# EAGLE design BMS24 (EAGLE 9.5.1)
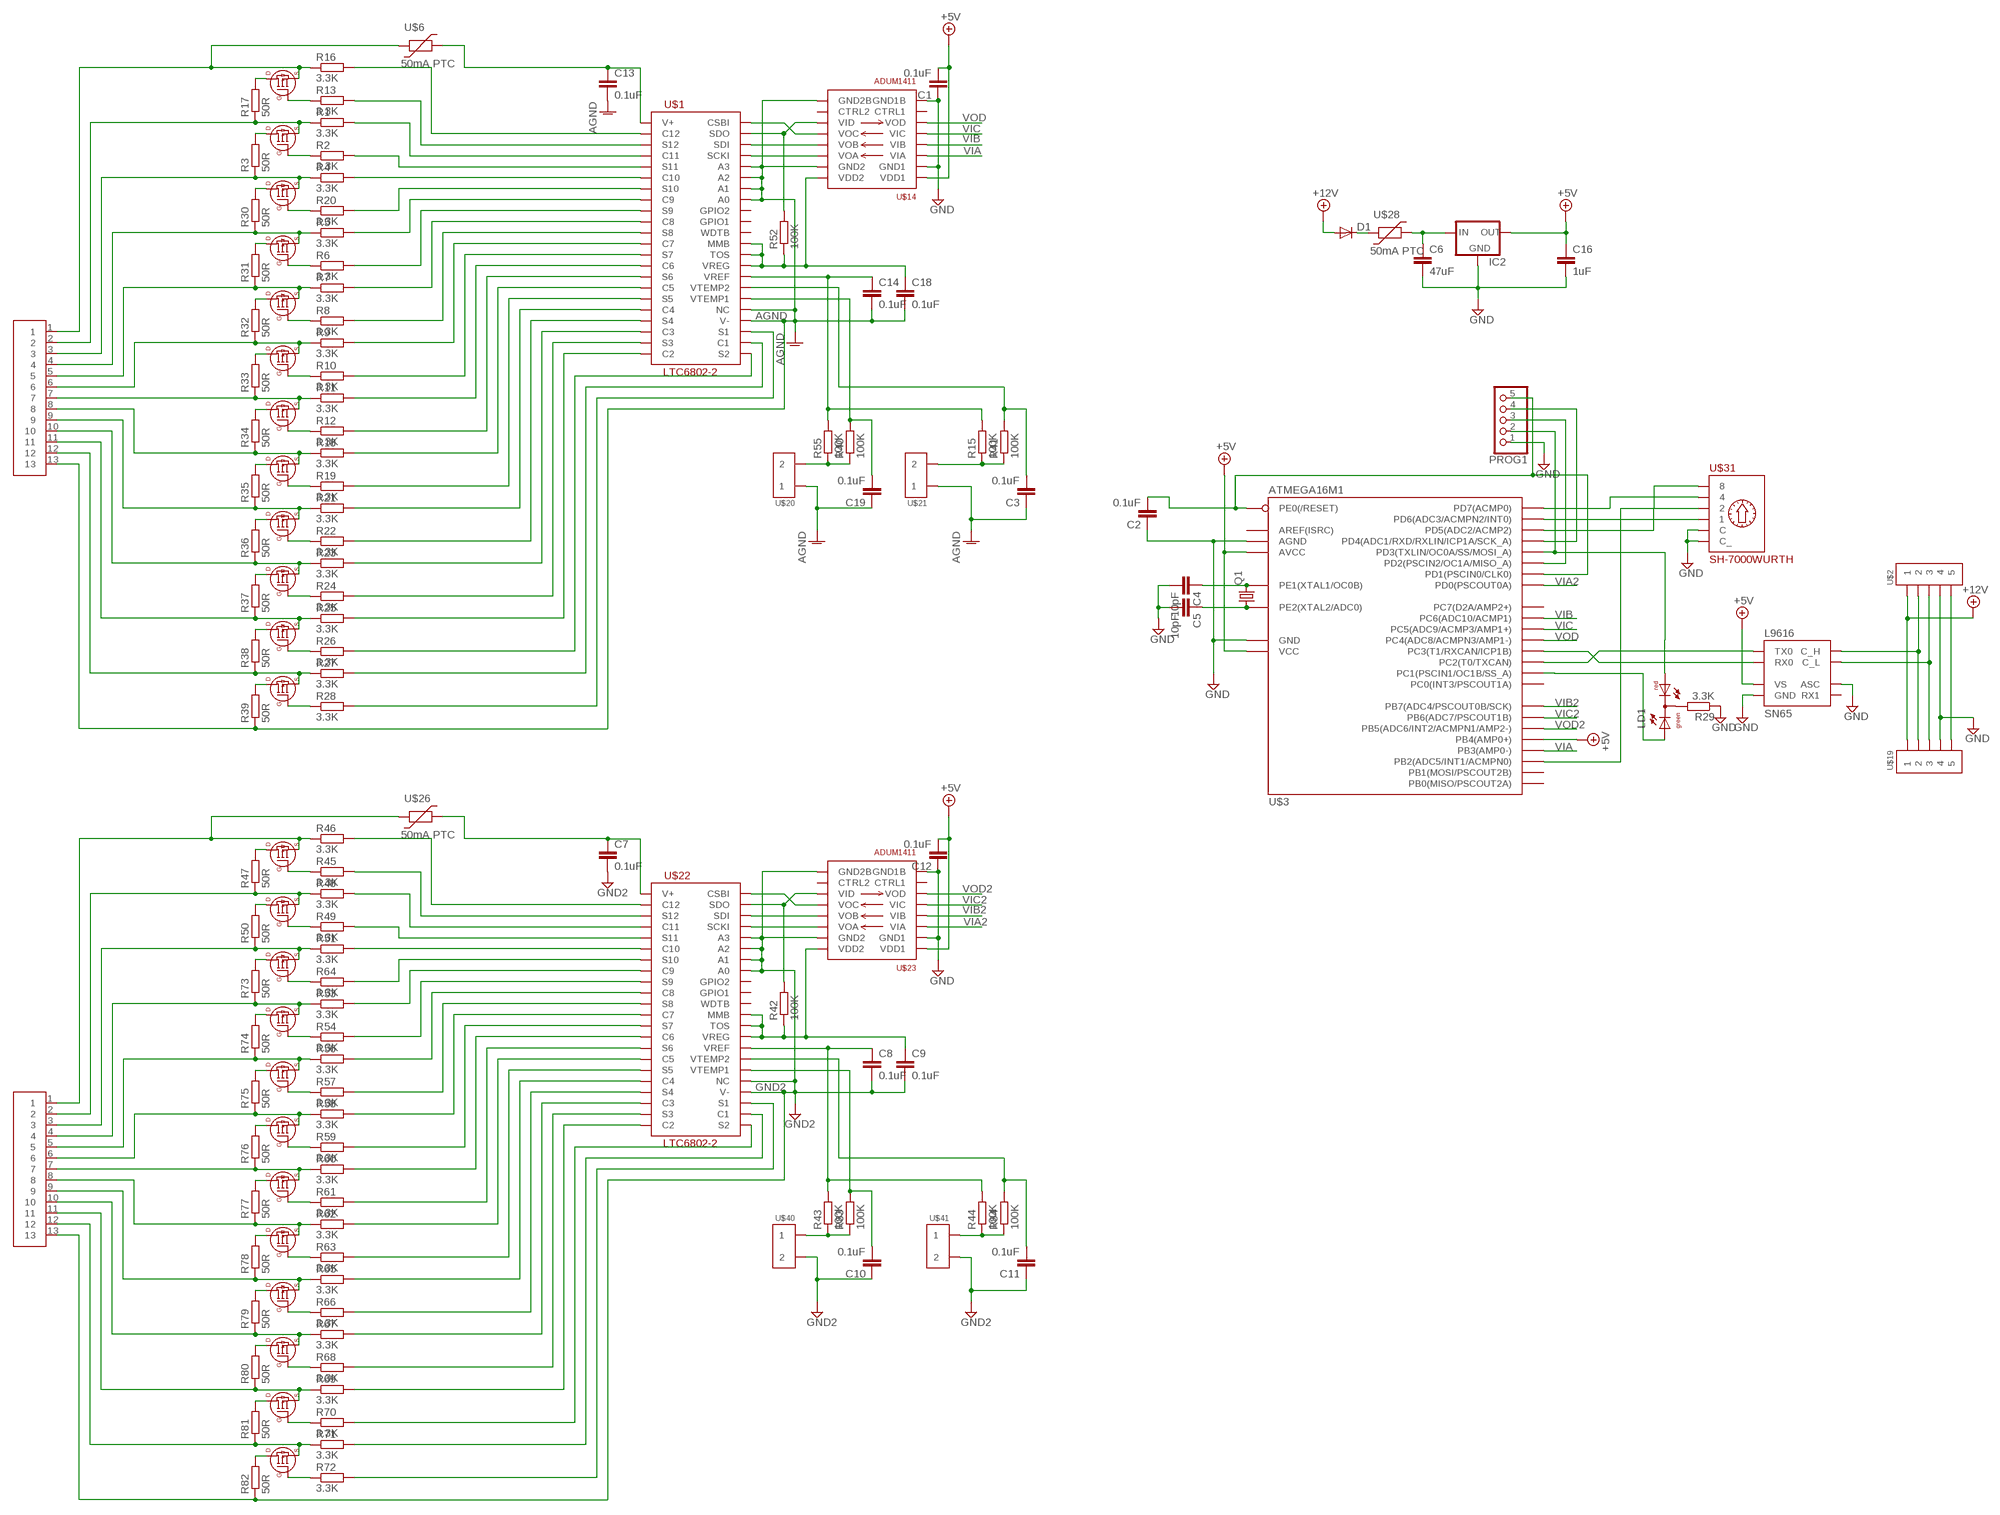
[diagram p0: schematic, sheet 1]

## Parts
C1  0.1uF  C-EUC0805  [C0805]
C2  0.1uF  C-EUC0805  [C0805]
C3  0.1uF  C-EUC0805  [C0805]
C4  10pF  C-EUC0805  [C0805]
C5  10pF  C-EUC0805  [C0805]
C6  47uF  C-EUC1206  [C1206]
C7  0.1uF  C-EUC0805  [C0805]
C8  0.1uF  C-EUC0805  [C0805]
C9  0.1uF  C-EUC0805  [C0805]
C10  0.1uF  C-EUC0805  [C0805]
C11  0.1uF  C-EUC0805  [C0805]
C12  0.1uF  C-EUC0805  [C0805]
C13  0.1uF  C-EUC0805  [C0805]
C14  0.1uF  C-EUC0805  [C0805]
C16  1uF  C-EUC0805  [C0805]
C18  0.1uF  C-EUC0805  [C0805]
C19  0.1uF  C-EUC0805  [C0805]
D1  DIODE-SOD123  [SOD123]
IC2  78LXXSOT89  [SOT89R]
LD1  DUOLED-RG-C  [DUOLED-C-5MM]
PROG1  PINHD-1X5  [1X05]
Q1  CRYSTALCTS406  [CTS406]
R1  3.3K  R-EU_R0805  [R0805]
R2  3.3K  R-EU_R0805  [R0805]
R3  50R  R-EU_R2512  [R2512]
R4  3.3K  R-EU_R0805  [R0805]
R5  3.3K  R-EU_R0805  [R0805]
R6  3.3K  R-EU_R0805  [R0805]
R7  3.3K  R-EU_R0805  [R0805]
R8  3.3K  R-EU_R0805  [R0805]
R9  3.3K  R-EU_R0805  [R0805]
R10  3.3K  R-EU_R0805  [R0805]
R11  3.3K  R-EU_R0805  [R0805]
R12  3.3K  R-EU_R0805  [R0805]
R13  3.3K  R-EU_R0805  [R0805]
R15  100K  R-EU_R0805  [R0805]
R16  3.3K  R-EU_R0805  [R0805]
R17  50R  R-EU_R2512  [R2512]
R18  3.3K  R-EU_R0805  [R0805]
R19  3.3K  R-EU_R0805  [R0805]
R20  3.3K  R-EU_R0805  [R0805]
R21  3.3K  R-EU_R0805  [R0805]
R22  3.3K  R-EU_R0805  [R0805]
R23  3.3K  R-EU_R0805  [R0805]
R24  3.3K  R-EU_R0805  [R0805]
R25  3.3K  R-EU_R0805  [R0805]
R26  3.3K  R-EU_R0805  [R0805]
R27  3.3K  R-EU_R0805  [R0805]
R28  3.3K  R-EU_R0805  [R0805]
R29  3.3K  R-EU_R0805  [R0805]
R30  50R  R-EU_R2512  [R2512]
R31  50R  R-EU_R2512  [R2512]
R32  50R  R-EU_R2512  [R2512]
R33  50R  R-EU_R2512  [R2512]
R34  50R  R-EU_R2512  [R2512]
R35  50R  R-EU_R2512  [R2512]
R36  50R  R-EU_R2512  [R2512]
R37  50R  R-EU_R2512  [R2512]
R38  50R  R-EU_R2512  [R2512]
R39  50R  R-EU_R2512  [R2512]
R40  100K  R-EU_R0805  [R0805]
R41  100K  R-EU_R0805  [R0805]
R42  100K  R-EU_R0805  [R0805]
R43  100K  R-EU_R0805  [R0805]
R44  100K  R-EU_R0805  [R0805]
R45  3.3K  R-EU_R0805  [R0805]
R46  3.3K  R-EU_R0805  [R0805]
R47  50R  R-EU_R2512  [R2512]
R48  3.3K  R-EU_R0805  [R0805]
R49  3.3K  R-EU_R0805  [R0805]
R50  50R  R-EU_R2512  [R2512]
R51  3.3K  R-EU_R0805  [R0805]
R52  100K  R-EU_R0805  [R0805]
R53  3.3K  R-EU_R0805  [R0805]
R54  3.3K  R-EU_R0805  [R0805]
R55  100K  R-EU_R0805  [R0805]
R56  3.3K  R-EU_R0805  [R0805]
R57  3.3K  R-EU_R0805  [R0805]
R58  3.3K  R-EU_R0805  [R0805]
R59  3.3K  R-EU_R0805  [R0805]
R60  3.3K  R-EU_R0805  [R0805]
R61  3.3K  R-EU_R0805  [R0805]
R62  3.3K  R-EU_R0805  [R0805]
R63  3.3K  R-EU_R0805  [R0805]
R64  3.3K  R-EU_R0805  [R0805]
R65  3.3K  R-EU_R0805  [R0805]
R66  3.3K  R-EU_R0805  [R0805]
R67  3.3K  R-EU_R0805  [R0805]
R68  3.3K  R-EU_R0805  [R0805]
R69  3.3K  R-EU_R0805  [R0805]
R70  3.3K  R-EU_R0805  [R0805]
R71  3.3K  R-EU_R0805  [R0805]
R72  3.3K  R-EU_R0805  [R0805]
R73  50R  R-EU_R2512  [R2512]
R74  50R  R-EU_R2512  [R2512]
R75  50R  R-EU_R2512  [R2512]
R76  50R  R-EU_R2512  [R2512]
R77  50R  R-EU_R2512  [R2512]
R78  50R  R-EU_R2512  [R2512]
R79  50R  R-EU_R2512  [R2512]
R80  50R  R-EU_R2512  [R2512]
R81  50R  R-EU_R2512  [R2512]
R82  50R  R-EU_R2512  [R2512]
R83  100K  R-EU_R0805  [R0805]
R84  100K  R-EU_R0805  [R0805]
SN65  L9616  [SOIC8]
U$1  LTC6802-2  [SSOP-44]
U$2  MOLEX-39502-1005  [MOLEX-39502-1005]
U$3  ATMEGA16M1  [TQFP32]
U$4  SI2351DS  [SOT23]
U$5  SI2351DS  [SOT23]
U$6  50mA PTC  1206_POLYSWITCH  [1206]
U$7  SI2351DS  [SOT23]
U$8  SI2351DS  [SOT23]
U$9  SI2351DS  [SOT23]
U$10  SI2351DS  [SOT23]
U$11  SI2351DS  [SOT23]
U$12  SI2351DS  [SOT23]
U$13  SI2351DS  [SOT23]
U$14  ADUM1411  [SOIC16W]
U$15  SI2351DS  [SOT23]
U$16  SI2351DS  [SOT23]
U$17  SI2351DS  [SOT23]
U$18  MOLEX_TERM_BLOCK_13  [MOLEX_TERM_BLOCK_13]
U$19  MOLEX-39502-1005  [MOLEX-39502-1005]
U$20  MOLEX-39502-1002  [MOLEX-39502-1002]
U$21  MOLEX-39502-1002  [MOLEX-39502-1002]
U$22  LTC6802-2  [SSOP-44]
U$23  ADUM1411  [SOIC16W]
U$24  SI2351DS  [SOT23]
U$25  SI2351DS  [SOT23]
U$26  50mA PTC  1206_POLYSWITCH  [1206]
U$27  SI2351DS  [SOT23]
U$28  50mA PTC  1206_POLYSWITCH  [1206]
U$29  SI2351DS  [SOT23]
U$30  SI2351DS  [SOT23]
U$31  SH-7000WURTH  [WS-ROTV]
U$32  SI2351DS  [SOT23]
U$33  SI2351DS  [SOT23]
U$34  SI2351DS  [SOT23]
U$35  SI2351DS  [SOT23]
U$36  SI2351DS  [SOT23]
U$37  SI2351DS  [SOT23]
U$38  SI2351DS  [SOT23]
U$39  MOLEX_TERM_BLOCK_13  [MOLEX_TERM_BLOCK_13]
U$40  MOLEX-39502-1002  [MOLEX-39502-1002]
U$41  MOLEX-39502-1002  [MOLEX-39502-1002]

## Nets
+5V: C1.2 C12.2 C16.1 IC2.2(OUT) SN65.P$3(VS) U$3.4(VCC) U$3.19(AVCC) U$3.24(PB4(AMP0+)) U$14.1(VDD1) U$23.1(VDD1)
+12V: D1.A U$2.1 U$19.1
AGND: C3.1 C13.2 C14.2 C18.2 C19.1 R39.1 U$1.26(V-) U$1.27(NC) U$1.37(A0) U$1.38(A1) U$1.39(A2) U$1.40(A3) U$14.9(GND2B) U$14.15(GND2) U$18.13 U$20.1 U$21.1
GND: C1.1 C2.1 C4.2 C5.2 C6.2 C12.1 C16.2 IC2.4(GND) PROG1.1 R29.1 SN65.P$2(GND) SN65.P$8(ASC) U$2.4 U$3.5(GND) U$3.20(AGND) U$14.2(GND1) U$14.8(GND1B) U$19.4 U$23.2(GND1) U$23.8(GND1B) U$31.C U$31.C2(C_)
GND2: C7.2 C8.2 C9.2 C10.1 C11.1 R82.1 U$22.26(V-) U$22.27(NC) U$22.37(A0) U$22.38(A1) U$22.39(A2) U$22.40(A3) U$23.9(GND2B) U$23.15(GND2) U$39.13 U$40.2 U$41.2
N$1: D1.C U$28.P$1
N$2: R16.2 U$1.2(C12)
N$3: R13.2 U$1.3(S12)
N$4: R3.2 U$5.P$3(D)
N$5: R1.2 U$1.4(C11)
N$6: R1.1 R17.1 U$5.P$2(S) U$18.2
N$7: U$1.42(SDI) U$14.13(VOB)
N$8: R3.1 R4.1 U$7.P$2(S) U$18.3
N$9: R4.2 U$1.6(C10)
N$10: R26.2 U$1.23(S2)
N$11: U$1.41(SCKI) U$14.14(VOA)
N$12: R27.2 U$1.24(C1)
N$13: R28.2 U$1.25(S1)
N$14: R2.2 U$1.5(S11)
N$15: R52.2 U$1.43(SDO) U$14.11(VID)
N$16: U$1.44(CSBI) U$14.12(VOC)
N$17: R2.1 U$5.P$1(G)
N$18: R30.2 U$7.P$3(D)
N$19: C2.2 PROG1.5 U$3.31(PE0(/RESET)) U$3.32(PD1(PSCIN0/CLK0))
N$20: C6.1 IC2.1(IN) U$28.P$2
N$21: R5.2 U$1.8(C9)
N$22: R7.2 U$1.10(C8)
N$23: R9.2 U$1.12(C7)
N$24: R11.2 U$1.14(C6)
N$25: C18.1 R52.1 U$1.31(VREG) U$1.32(TOS) U$1.33(MMB) U$14.16(VDD2)
N$26: R18.2 U$1.16(C5)
N$27: R21.2 U$1.18(C4)
N$28: R23.2 U$1.20(C3)
N$29: R25.2 U$1.22(C2)
N$30: U$3.16(PB2(ADC5/INT1/ACMPN0)) U$31.2
N$31: R5.1 R30.1 U$8.P$2(S) U$18.4
N$32: LD1.AR PROG1.2 U$3.2(PD3(TXLIN/OC0A/SS/MOSI_A))
N$33: PROG1.3 U$3.1(PD2(PSCIN2/OC1A/MISO_A))
N$34: PROG1.4 U$3.12(PD4(ADC1/RXD/RXLIN/ICP1A/SCK_A))
N$35: U$22.42(SDI) U$23.13(VOB)
N$36: SN65.P$4(RX0) U$3.7(PC3(T1/RXCAN/ICP1B))
N$37: SN65.P$1(TX0) U$3.6(PC2(T0/TXCAN))
N$38: SN65.P$7(C_H) U$2.2 U$19.2
N$39: SN65.P$6(C_L) U$2.3 U$19.3
N$40: LD1.C R29.2
N$41: LD1.AX(AG) U$3.3(PC1(PSCIN1/OC1B/SS_A))
N$42: U$3.15(PD7(ACMP0)) U$31.4
N$44: U$3.14(PD6(ADC3/ACMPN2/INT0)) U$31.1
N$45: U$3.13(PD5(ADC2/ACMP2)) U$31.8
N$46: C3.2 R41.2 U$1.29(VTEMP2)
N$47: U$2.5 U$19.5
N$48: C4.1 Q1.3 U$3.10(PE1(XTAL1/OC0B))
N$49: C5.1 Q1.1 U$3.11(PE2(XTAL2/ADC0))
N$50: R17.2 U$4.P$3(D)
N$51: R16.1 U$4.P$2(S) U$6.P$1 U$18.1
N$52: R13.1 U$4.P$1(G)
N$53: R7.1 R31.1 U$9.P$2(S) U$18.5
N$54: R31.2 U$8.P$3(D)
N$55: R6.1 U$8.P$1(G)
N$56: R20.1 U$7.P$1(G)
N$57: R8.1 U$9.P$1(G)
N$58: R10.1 U$10.P$1(G)
N$59: R12.1 U$11.P$1(G)
N$60: R28.1 U$17.P$1(G)
N$61: R19.1 U$12.P$1(G)
N$62: R22.1 U$13.P$1(G)
N$63: R24.1 U$15.P$1(G)
N$64: R26.1 U$16.P$1(G)
N$65: R27.1 R38.1 U$17.P$2(S) U$18.12
N$66: C14.1 R15.2 R55.2 U$1.30(VREF)
N$67: C19.2 R40.2 U$1.28(VTEMP1)
N$69: R25.1 R37.1 U$16.P$2(S) U$18.11
N$70: R23.1 R36.1 U$15.P$2(S) U$18.10
N$71: R38.2 U$16.P$3(D)
N$72: R39.2 U$17.P$3(D)
N$73: R37.2 U$15.P$3(D)
N$74: R21.1 R35.1 U$13.P$2(S) U$18.9
N$75: R36.2 U$13.P$3(D)
N$76: R18.1 R34.1 U$12.P$2(S) U$18.8
N$77: R35.2 U$12.P$3(D)
N$78: R11.1 R33.1 U$11.P$2(S) U$18.7
N$79: R9.1 R32.1 U$10.P$2(S) U$18.6
N$80: R33.2 U$10.P$3(D)
N$81: R34.2 U$11.P$3(D)
N$82: R32.2 U$9.P$3(D)
N$83: R24.2 U$1.21(S3)
N$84: R22.2 U$1.19(S4)
N$85: R40.1 R55.1 U$20.2
N$86: R15.1 R41.1 U$21.2
N$87: R20.2 U$1.7(S10)
N$88: R6.2 U$1.9(S9)
N$89: R8.2 U$1.11(S8)
N$90: R10.2 U$1.13(S7)
N$91: R12.2 U$1.15(S6)
N$92: U$22.41(SCKI) U$23.14(VOA)
N$93: R19.2 U$1.17(S5)
N$94: R42.2 U$22.43(SDO) U$23.11(VID)
N$95: U$22.44(CSBI) U$23.12(VOC)
N$96: C9.1 R42.1 U$22.31(VREG) U$22.32(TOS) U$22.33(MMB) U$23.16(VDD2)
N$97: C8.1 R43.2 R44.2 U$22.30(VREF)
N$98: C10.2 R83.2 U$22.28(VTEMP1)
N$99: R70.2 U$22.23(S2)
N$100: R71.2 U$22.24(C1)
N$101: R72.2 U$22.25(S1)
N$102: C11.2 R84.2 U$22.29(VTEMP2)
N$103: R47.2 U$24.P$3(D)
N$104: R45.1 U$24.P$1(G)
N$105: R46.1 U$24.P$2(S) U$26.P$1 U$39.1
N$106: R46.2 U$22.2(C12)
N$107: R45.2 U$22.3(S12)
N$108: R48.2 U$22.4(C11)
N$109: R47.1 R48.1 U$25.P$2(S) U$39.2
N$110: R50.2 U$25.P$3(D)
N$111: R50.1 R51.1 U$27.P$2(S) U$39.3
N$112: R51.2 U$22.6(C10)
N$113: R49.2 U$22.5(S11)
N$114: R49.1 U$25.P$1(G)
N$115: R73.2 U$27.P$3(D)
N$116: R53.2 U$22.8(C9)
N$117: R56.2 U$22.10(C8)
N$118: R58.2 U$22.12(C7)
N$119: R60.2 U$22.14(C6)
N$120: R62.2 U$22.16(C5)
N$121: R65.2 U$22.18(C4)
N$122: R67.2 U$22.20(C3)
N$123: R69.2 U$22.22(C2)
N$124: R53.1 R73.1 U$29.P$2(S) U$39.4
N$125: R56.1 R74.1 U$30.P$2(S) U$39.5
N$126: R74.2 U$29.P$3(D)
N$127: R54.1 U$29.P$1(G)
N$128: R64.1 U$27.P$1(G)
N$129: R57.1 U$30.P$1(G)
N$130: R59.1 U$32.P$1(G)
N$131: R61.1 U$33.P$1(G)
N$132: R72.1 U$38.P$1(G)
N$133: R63.1 U$34.P$1(G)
N$134: R66.1 U$35.P$1(G)
N$135: R68.1 U$36.P$1(G)
N$136: R70.1 U$37.P$1(G)
N$137: R71.1 R81.1 U$38.P$2(S) U$39.12
N$138: R69.1 R80.1 U$37.P$2(S) U$39.11
N$139: R67.1 R79.1 U$36.P$2(S) U$39.10
N$140: R81.2 U$37.P$3(D)
N$141: R82.2 U$38.P$3(D)
N$142: R80.2 U$36.P$3(D)
N$143: R65.1 R78.1 U$35.P$2(S) U$39.9
N$144: R79.2 U$35.P$3(D)
N$145: R62.1 R77.1 U$34.P$2(S) U$39.8
N$146: R78.2 U$34.P$3(D)
N$147: R60.1 R76.1 U$33.P$2(S) U$39.7
N$148: R58.1 R75.1 U$32.P$2(S) U$39.6
N$149: R76.2 U$32.P$3(D)
N$150: R77.2 U$33.P$3(D)
N$151: R75.2 U$30.P$3(D)
N$152: R64.2 U$22.7(S10)
N$153: R54.2 U$22.9(S9)
N$154: R57.2 U$22.11(S8)
N$155: R59.2 U$22.13(S7)
N$156: R61.2 U$22.15(S6)
N$157: R63.2 U$22.17(S5)
N$158: R66.2 U$22.19(S4)
N$159: R68.2 U$22.21(S3)
N$160: R43.1 R83.1 U$40.1
N$161: R44.1 R84.1 U$41.1
V+: C13.1 U$1.1(V+) U$6.P$2
V+1: C7.1 U$22.1(V+) U$26.P$2
VIA: U$3.23(PB3(AMP0-)) U$14.3(VIA)
VIA2: U$3.29(PD0(PSCOUT0A)) U$23.3(VIA)
VIB: U$3.22(PC6(ADC10/ACMP1)) U$14.4(VIB)
VIB2: U$3.28(PB7(ADC4/PSCOUT0B/SCK)) U$23.4(VIB)
VIC: U$3.18(PC5(ADC9/ACMP3/AMP1+)) U$14.5(VIC)
VIC2: U$3.27(PB6(ADC7/PSCOUT1B)) U$23.5(VIC)
VOD: U$3.17(PC4(ADC8/ACMPN3/AMP1-)) U$14.6(VOD)
VOD2: U$3.26(PB5(ADC6/INT2/ACMPN1/AMP2-)) U$23.6(VOD)
Unconnected: SN65.P$5(RX1) U$1.34(WDTB) U$1.35(GPIO1) U$1.36(GPIO2) U$3.8(PB0(MISO/PSCOUT2A)) U$3.9(PB1(MOSI/PSCOUT2B)) U$3.21(AREF(ISRC)) U$3.25(PC7(D2A/AMP2+)) U$3.30(PC0(INT3/PSCOUT1A)) U$14.7(CTRL1) U$14.10(CTRL2) U$22.34(WDTB) U$22.35(GPIO1) U$22.36(GPIO2) U$23.7(CTRL1) U$23.10(CTRL2)

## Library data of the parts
C1-C14 C16 C18 C19 = resistor:C-EU: CAPACITOR, European symbol
D1 = diode:DIODE-: DIODE
IC2 = v-reg:78LXX: VOLTAGE REGULATOR
LD1 = led:DUOLED-RG-C: DUO LED 2 colors (red/green), 5 mm, round, common Cathode www.ligitek.com or other producers.
PROG1 = pinhead:PINHD-1X5: PIN HEADER
Q1 = crystal:CRYSTAL: CRYSTAL
R1-R13 R15-R84 = resistor:R-EU_: RESISTOR, European symbol
SN65 = Ians parts:L9616
U$1 U$22 = Ians parts:LTC6802-2
U$2 U$19 = Ians parts:MOLEX-39502-1005
U$3 = Ians parts:ATMEGA16M1
U$4 U$5 U$7-U$13 U$15-U$17 U$24 U$25 U$27 U$29 U$30 U$32-U$38 = Ians parts:SI2351DS
U$6 U$26 U$28 = Ians parts:1206_POLYSWITCH
U$14 U$23 = Ians parts:ADUM1411
U$18 U$39 = Ians parts:MOLEX_TERM_BLOCK_13
U$20 U$21 U$40 U$41 = Ians parts:MOLEX-39502-1002
U$31 = Ians parts:SH-7000

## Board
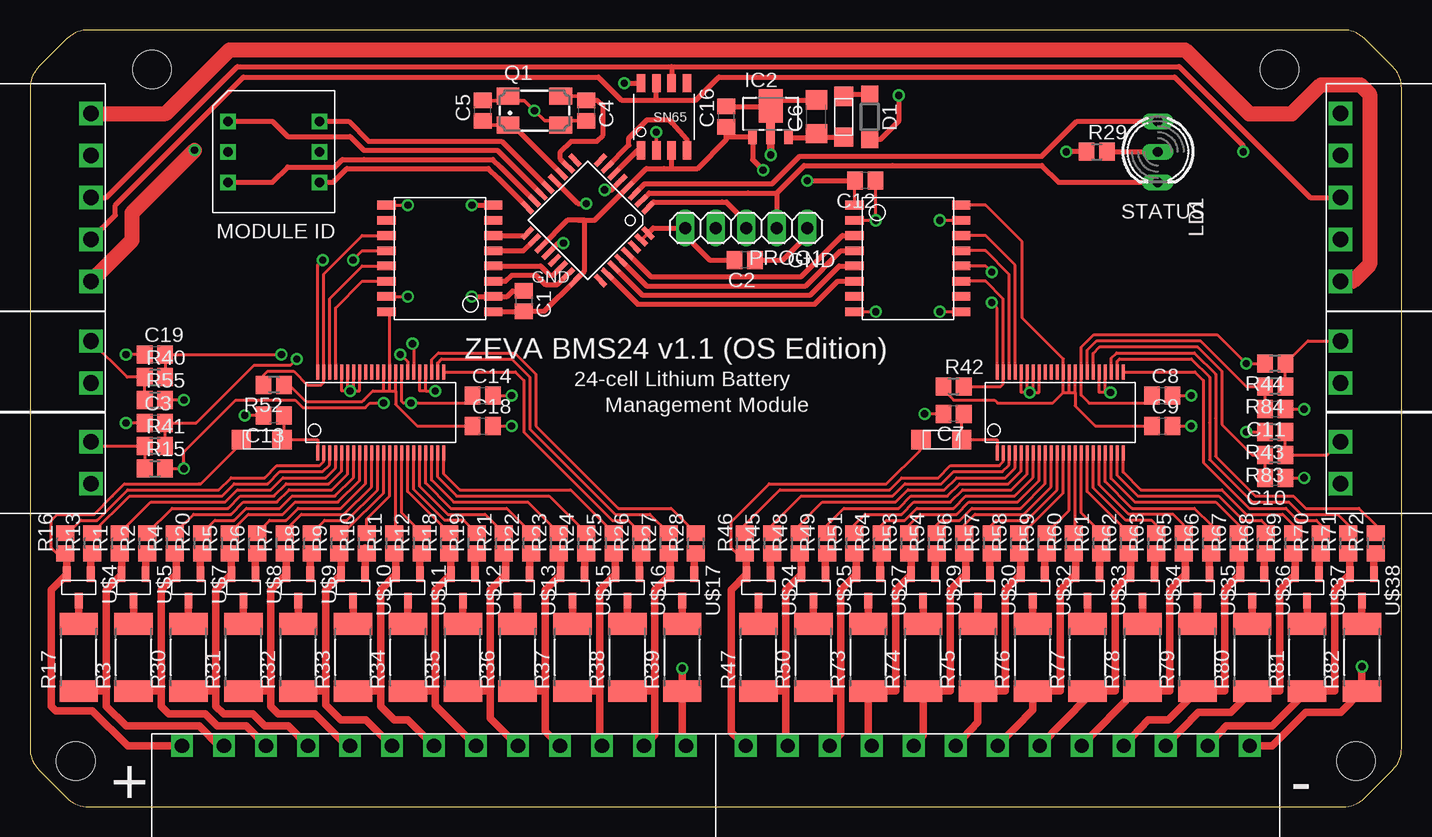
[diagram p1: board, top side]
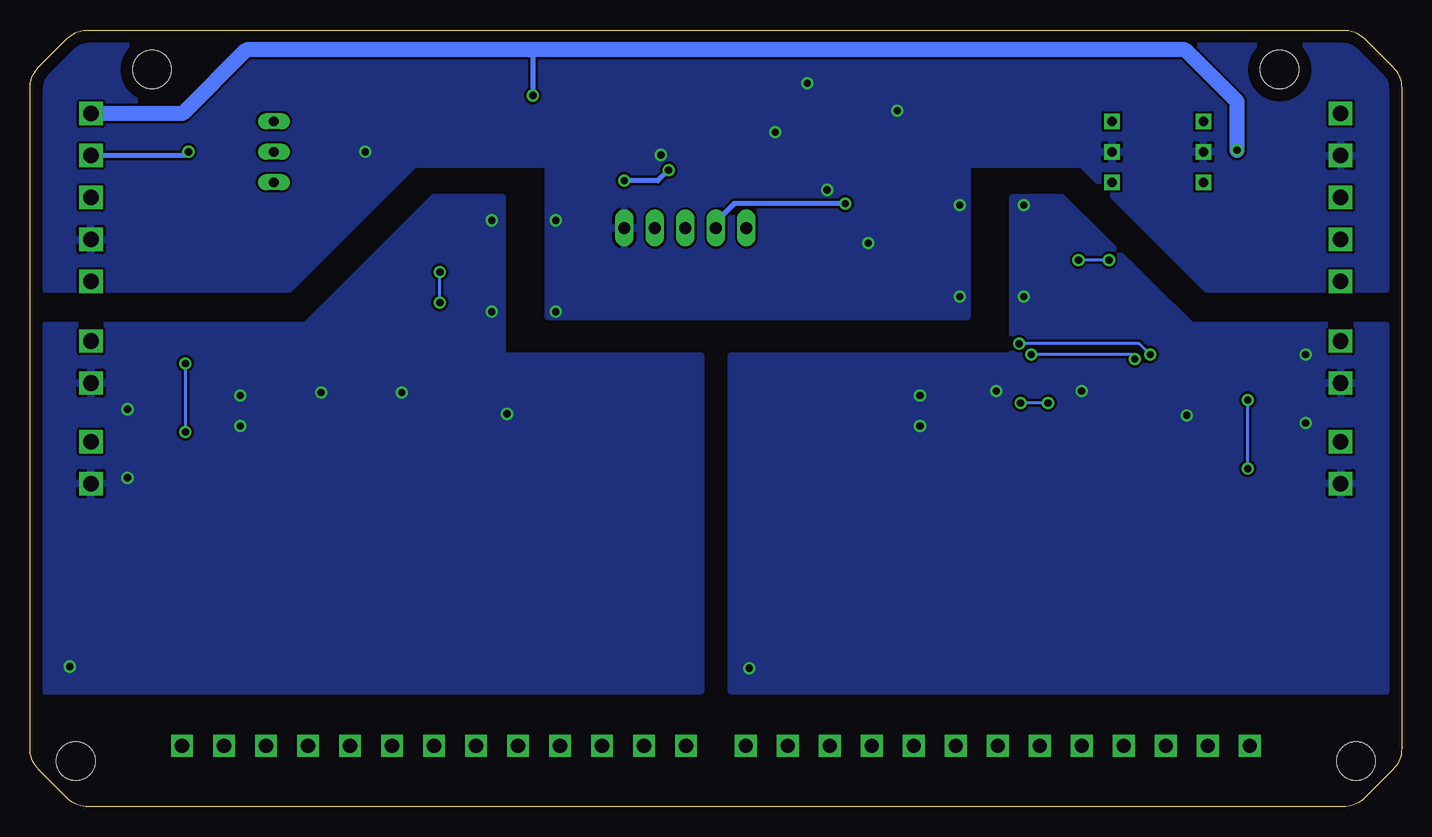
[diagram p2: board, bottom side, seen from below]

Size 114.3 x 64.77 mm. Coordinates in mm from the lower left corner, seen from the top.
Outline: 4.86,64.77 arc45 3.07,64.03 0.74,61.7 arc45 0,59.91 0,4.86 arc45 0.74,3.07 3.07,0.74 arc45 4.86,0 109.44,0 arc45 111.23,0.74 113.56,3.07 arc45 114.3,4.86 114.3,59.91 arc45 113.56,61.7 111.23,64.03 arc45 109.44,64.77 4.86,64.77
Copper layers (1*16): Top 0.035mm / dielectric 1.5mm / Bottom 0.035mm
Design rules "default *": minimum track width 10mil, minimum drill 10mil, track to track 8mil, track to pad 8mil, pad to pad 8mil, via to via 8mil, smd to smd 8mil, copper to edge 40mil, drill to drill 8mil, minimum pad ring 10mil, minimum via ring 8mil, stop-mask expansion 4mil, vias tented up to drill 0mil, thermal gap 10mil
Holes 3.2 mm at 3.81,3.81 110.49,3.81 10.16,61.47 104.14,61.47

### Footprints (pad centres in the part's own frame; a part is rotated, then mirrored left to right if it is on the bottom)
C0805 = smd 1.3 x 1.5: 1 -0.85,0; 2 0.85,0
C1206 = smd 1.6 x 1.8: 1 -1.4,0; 2 1.4,0
SOD123 = smd 1.4 x 1.4: A 1.9,0; C -1.9,0
SOT89R = smd 0.7 x 1.1: 1 1.5,-1.75; 2 -1.5,-1.75 | smd 0.7 x 1.8: 3 0,-1.4 | smd 2 x 2.8: 4 0,0.9
DUOLED-C-5MM = drill 0.813 long: AR 2.54,0; AX -2.54,0; C 0,0
1X05 = drill 1.016 long: 1 -5.08,0; 2 -2.54,0; 3 0,0; 4 2.54,0; 5 5.08,0
CTS406 = smd 1.9 x 1.4: 1 -2.2,-1.2; 2 2.2,-1.2; 3 2.2,1.2; 4 -2.2,1.2
R0805 = smd 1.3 x 1.5: 1 -0.85,0; 2 0.85,0
R2512 = smd 1.8 x 3.2: 1 -2.8,0; 2 2.8,0
SOIC8 = smd 1.524 x 0.711: P$1 -2.794,1.905; P$2 -2.794,0.635; P$3 -2.794,-0.635; P$4 -2.794,-1.905; P$5 2.794,-1.905; P$6 2.794,-0.635; P$7 2.794,0.635; P$8 2.794,1.905
SSOP-44 = smd 1.25 x 0.25: 1 -3.375,5.25; 2 -3.375,4.75; 3 -3.375,4.25; 4 -3.375,3.75; 5 -3.375,3.25; 6 -3.375,2.75; 7 -3.375,2.25; 8 -3.375,1.75; 9 -3.375,1.25; 10 -3.375,0.75; 11 -3.375,0.25; 12 -3.375,-0.25; 13 -3.375,-0.75; 14 -3.375,-1.25; 15 -3.375,-1.75; 16 -3.375,-2.25; 17 -3.375,-2.75; 18 -3.375,-3.25; 19 -3.375,-3.75; 20 -3.375,-4.25; 21 -3.375,-4.75; 22 -3.375,-5.25; 23 3.375,-5.25; 24 3.375,-4.75; 25 3.375,-4.25; 26 3.375,-3.75; 27 3.375,-3.25; 28 3.375,-2.75; 29 3.375,-2.25; 30 3.375,-1.75; 31 3.375,-1.25; 32 3.375,-0.75; 33 3.375,-0.25; 34 3.375,0.25; 35 3.375,0.75; 36 3.375,1.25; 37 3.375,1.75; 38 3.375,2.25; 39 3.375,2.75; 40 3.375,3.25; 41 3.375,3.75; 42 3.375,4.25; 43 3.375,4.75; 44 3.375,5.25
MOLEX-39502-1005 = drill 1.3 square: 1 -7,0; 2 -3.5,0; 3 0,0; 4 3.5,0; 5 7,0
TQFP32 = smd 1.2 x 0.4: 1 -4.3,2.8; 2 -4.3,2; 3 -4.3,1.2; 4 -4.3,0.4; 5 -4.3,-0.4; 6 -4.3,-1.2; 7 -4.3,-2; 8 -4.3,-2.8; 17 4.3,-2.8; 18 4.3,-2; 19 4.3,-1.2; 20 4.3,-0.4; 21 4.3,0.4; 22 4.3,1.2; 23 4.3,2; 24 4.3,2.8 | smd 0.4 x 1.2: 9 -2.8,-4.3; 10 -2,-4.3; 11 -1.2,-4.3; 12 -0.4,-4.3; 13 0.4,-4.3; 14 1.2,-4.3; 15 2,-4.3; 16 2.8,-4.3; 25 2.8,4.3; 26 2,4.3; 27 1.2,4.3; 28 0.4,4.3; 29 -0.4,4.3; 30 -1.2,4.3; 31 -2,4.3; 32 -2.8,4.3
SOT23 = smd 1.27 x 0.635: P$1 -1.1,1; P$2 -1.1,-1; P$3 1.1,0
1206 = smd 1.6 x 1.6: P$1 -1.7,0; P$2 1.7,0
SOIC16W = smd 1.524 x 0.711: 1 -4.445,4.445; 2 -4.445,3.175; 3 -4.445,1.905; 4 -4.445,0.635; 5 -4.445,-0.635; 6 -4.445,-1.905; 7 -4.445,-3.175; 8 -4.445,-4.445; 9 4.445,-4.445; 10 4.445,-3.175; 11 4.445,-1.905; 12 4.445,-0.635; 13 4.445,0.635; 14 4.445,1.905; 15 4.445,3.175; 16 4.445,4.445
MOLEX_TERM_BLOCK_13 = drill 1.2 square: 1 -21,0; 2 -17.5,0; 3 -14,0; 4 -10.5,0; 5 -7,0; 6 -3.5,0; 7 0,0; 8 3.5,0; 9 7,0; 10 10.5,0; 11 14,0; 12 17.5,0; 13 21,0
MOLEX-39502-1002 = drill 1.3 square: 1 -1.75,0; 2 1.75,0
WS-ROTV = drill 0.8 square: 1 -3.81,2.54; 2 3.81,-2.54; 4 -3.81,-2.54; 8 3.81,2.54; C -3.81,0; C2 3.81,0

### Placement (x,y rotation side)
C1  41.15,42.16 270 top
C2  59.56,45.59 180 top
C3  10.41,32 0 top
C4  46.35,58.04 270 top
C5  37.72,58.04 90 top
C6  65.53,57.53 90 top
C7  76.96,32.77 180 top
C8  94.36,34.29 0 top
C9  94.36,31.75 0 top
C10  103.76,27.43 180 top
C11  103.76,33.15 180 top
C12  69.6,52.2 180 top
C13  20.32,32.64 180 top
C14  37.72,34.29 0 top
C16  58.04,57.53 90 top
C18  37.72,31.75 0 top
C19  10.41,37.72 0 top
D1  69.98,57.53 270 top
IC2  61.72,57.53 0 top
LD1  93.98,54.61 270 top
PROG1  59.69,48.26 180 top
Q1  42.04,58.04 0 top
R1  7.49,21.97 90 top
R2  9.78,21.97 90 top
R3  8.64,12.45 90 top
R4  12.06,21.97 90 top
R5  16.64,21.97 90 top
R6  18.92,21.97 90 top
R7  21.21,21.97 90 top
R8  23.5,21.97 90 top
R9  25.78,21.97 90 top
R10  28.07,21.97 90 top
R11  30.35,21.97 90 top
R12  32.64,21.97 90 top
R13  5.21,21.97 90 top
R15  10.41,28.19 0 top
R16  2.92,21.97 90 top
R17  4.06,12.45 90 top
R18  34.92,21.97 90 top
R19  37.21,21.97 90 top
R20  14.35,21.97 90 top
R21  39.5,21.97 90 top
R22  41.78,21.97 90 top
R23  44.07,21.97 90 top
R24  46.35,21.97 90 top
R25  48.64,21.97 90 top
R26  50.93,21.97 90 top
R27  53.21,21.97 90 top
R28  55.5,21.97 90 top
R29  88.9,54.61 0 top
R30  13.21,12.45 90 top
R31  17.78,12.45 90 top
R32  22.35,12.45 90 top
R33  26.92,12.45 90 top
R34  31.5,12.45 90 top
R35  36.07,12.45 90 top
R36  40.64,12.45 90 top
R37  45.21,12.45 90 top
R38  49.78,12.45 90 top
R39  54.36,12.45 90 top
R40  10.41,35.81 0 top
R41  10.41,30.1 0 top
R42  76.96,35.05 0 top
R43  103.76,31.24 180 top
R44  103.76,36.96 180 top
R45  61.85,21.97 90 top
R46  59.56,21.97 90 top
R47  60.71,12.45 90 top
R48  64.14,21.97 90 top
R49  66.42,21.97 90 top
R50  65.28,12.45 90 top
R51  68.71,21.97 90 top
R52  20.32,35.18 180 top
R53  73.28,21.97 90 top
R54  75.56,21.97 90 top
R55  10.41,33.91 0 top
R56  77.85,21.97 90 top
R57  80.14,21.97 90 top
R58  82.42,21.97 90 top
R59  84.71,21.97 90 top
R60  87,21.97 90 top
R61  89.28,21.97 90 top
R62  91.57,21.97 90 top
R63  93.85,21.97 90 top
R64  70.99,21.97 90 top
R65  96.14,21.97 90 top
R66  98.42,21.97 90 top
R67  100.71,21.97 90 top
R68  103,21.97 90 top
R69  105.28,21.97 90 top
R70  107.57,21.97 90 top
R71  109.86,21.97 90 top
R72  112.14,21.97 90 top
R73  69.85,12.45 90 top
R74  74.42,12.45 90 top
R75  78.99,12.45 90 top
R76  83.57,12.45 90 top
R77  88.14,12.45 90 top
R78  92.71,12.45 90 top
R79  97.28,12.45 90 top
R80  101.85,12.45 90 top
R81  106.43,12.45 90 top
R82  111,12.45 90 top
R83  103.76,29.34 180 top
R84  103.76,35.05 180 top
SN65  52.83,57.53 90 top
U$1  29.21,32.89 90 top
U$2  5.08,50.8 90 top
U$3  46.48,48.9 225 top
U$4  4.06,18.29 270 top
U$5  8.64,18.29 270 top
U$6  19.3,30.61 0 top
U$7  13.21,18.29 270 top
U$8  17.78,18.29 270 top
U$9  22.35,18.29 270 top
U$10  26.92,18.29 270 top
U$11  31.5,18.29 270 top
U$12  36.07,18.29 270 top
U$13  40.64,18.29 270 top
U$14  34.16,45.72 180 top
U$15  45.21,18.29 270 top
U$16  49.78,18.29 270 top
U$17  54.36,18.29 270 top
U$18  33.66,5.08 0 top
U$19  109.22,50.8 270 top
U$20  5.08,37.08 90 top
U$21  5.08,28.7 90 top
U$22  85.85,32.89 90 top
U$23  73.15,45.72 0 top
U$24  60.71,18.29 270 top
U$25  65.28,18.29 270 top
U$26  75.95,30.61 0 top
U$27  69.85,18.29 270 top
U$28  67.82,57.53 270 top
U$29  74.42,18.29 270 top
U$30  78.99,18.29 270 top
U$31  20.32,54.61 0 top
U$32  83.57,18.29 270 top
U$33  88.14,18.29 270 top
U$34  92.71,18.29 270 top
U$35  97.28,18.29 270 top
U$36  101.85,18.29 270 top
U$37  106.43,18.29 270 top
U$38  111,18.29 270 top
U$39  80.64,5.08 0 top
U$40  109.22,28.7 270 top
U$41  109.22,37.08 270 top

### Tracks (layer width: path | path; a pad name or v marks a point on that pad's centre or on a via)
+5V  (via drill 0.6)
  Top 0.254: U$23.1 68.71,52.16 C12.2
  Top 0.406: U$14.1 41.11,41.27 C1.2 42.86,41.31 U$3.24 46.23,44.68 46.23,47.24 46.23,48.9 45.72,48.9 | U$3.19 44.78,48.9 45.72,48.9 | 45.72,48.9 45.85,48.9 47.05,48.9 U$3.4 51.37,53.21 52.83,53.21 | 52.83,53.21 55.63,53.21 58.04,55.63 58.04,55.88 | 58.04,55.88 C16.1 | SN65.P$3 53.47,53.21 52.83,53.21 | 58.04,55.88 60.22,55.88 IC2.2 60.22,53.95 v61.09,53.09 | v64.77,52.2 C12.2
  Bottom 0.406: v64.77,52.2 61.98,52.2 v61.09,53.09
+12V  (via drill 0.6)
  Top 0.406: D1.A 70.87,55.63 72.39,57.15 v72.39,59.31
  Top 1.27: U$2.1 8.51,47.23 8.51,49.53 v13.72,54.74
  Bottom 0.406: v72.39,59.31 72.39,63.12 72.64,63.12
  Bottom 1.27: U$19.1 101.58,57.8 96.27,63.12 72.64,63.12 18.03,63.12 13.72,58.8 v13.72,54.74
AGND  (via drill 0.6)
  Top 0.254: 32.96,34.67 U$1.26 | 32.96,34.67 v33.78,34.67 | U$1.27 32.46,34.67 32.96,34.67 | U$1.37 27.46,34.67 v26.67,34.67 | U$1.38 26.96,34.67 v26.67,34.67 | U$1.39 26.46,34.67 v26.67,34.67 | U$1.40 25.96,34.67 v26.67,34.67 | C14.2 v40.13,34.29 | C18.2 v40.13,31.75 | C3.1 v8,32 | C19.1 v8,37.72 | C13.2 v17.91,32.64 | U$14.15 v31.5,42.55 | U$14.9 v31.5,50.16
  Top 0.61: v54.36,11.56 R39.1 54.36,5.38 U$18.13
  pour Bottom: 1.27,9.65 55.88,9.65 55.88,37.59 32.38,37.59 32.38,50.8 28.32,50.8 17.53,40.13 1.27,40.13
GND  (via drill 0.6)
  Top 0.254: U$23.2 v70.48,48.9 70.48,52.16 C12.1 | U$23.8 v70.48,41.27
  Top 0.305: SN65.P$2 v52.2,56.26 | C5.2 41.19,58.89 v42.04,58.04 42.89,57.19 C4.2
  Top 0.406: C1.1 40.22,43.01 39.75,42.55 U$14.2 v36.83,42.55 | v36.83,50.16 U$14.8 | U$3.20 44.01,46.99 v44.45,46.99 | v47.88,51.44 48.46,51.44 U$3.5 | C2.1 62.74,45.59 64.77,47.62 PROG1.1 | v49.53,60.33 SN65.P$8 | C6.2 62.22,58.93 IC2.4 61.67,58.38 C16.2 | R29.1 v86.36,54.61
  Top 0.61: IC2.4 v61.72,54.36
  pour Bottom: 36.2,40.89 36.2,53.59 26.67,53.59 16.26,43.18 1.27,43.18 1.27,63.5 113.03,63.5 113.03,43.18 92.71,43.18 82.3,53.59 71.12,53.59 71.12,40.89
GND2  (via drill 0.6)
  Top 0.254: U$22.39 83.1,34.54 v83.31,34.54 | U$22.40 82.6,34.54 v83.31,34.54 | U$22.38 83.6,34.54 v83.31,34.54 | U$22.37 84.1,34.54 v83.31,34.54 | C8.2 v96.77,34.29 | C9.2 v96.77,31.75 | U$22.26 89.6,34.54 v90.04,34.54 89.1,34.54 U$22.27 | C10.1 v106.17,27.43 | C11.1 v106.17,33.15 | C7.2 v74.55,32.77 | v75.82,41.27 U$23.9 | v75.82,48.9 U$23.15
  Top 0.61: v111,11.68 R82.1 109.23,7.87 106.3,7.87 103.5,5.08 U$39.13
  pour Bottom: 58.42,9.65 113.03,9.65 113.03,40.13 91.31,40.13 80.64,50.8 74.93,50.8 74.93,37.59 58.42,37.59
N$1
  Top 0.406: D1.C 68.02,59.43 U$28.P$1
N$2
  Top 0.254: U$1.2 24.46,28.78 24.13,28.45 20.57,28.45 19.56,27.43 16.76,27.43 15.75,26.42 8.13,26.42 5.59,23.88 4.23,23.88 3.17,22.82 R16.2
N$3
  Top 0.254: U$1.3 24.96,28.52 24.38,27.94 20.83,27.94 19.81,26.92 17.02,26.92 16,25.91 8.29,25.91 R13.2
N$4
  Top 0.61: R3.2 U$5.P$3
N$5
  Top 0.254: U$1.4 25.46,28.25 24.64,27.43 21.08,27.43 20.07,26.42 17.27,26.42 16.26,25.4 10.07,25.4 R1.2
N$6
  Top 0.61: 6.35,9.65 6.35,18.1 U$5.P$2 7.64,20.98 R1.1 | R17.1 6.35,9.65 | 6.35,9.65 6.35,8.38 8,6.73 8.38,6.73 14.1,6.73 15.75,5.08 U$18.2
N$7
  Top 0.254: U$1.42 24.96,42.36 27.69,45.09 U$14.13
N$8
  Top 0.61: 10.92,9.65 10.92,18.1 U$7.P$2 12.21,20.98 R4.1 | R3.1 10.92,9.65 | U$18.3 18,6.73 15.62,6.73 14.61,7.75 11.56,7.75 10.92,8.38 10.92,9.65
N$9
  Top 0.254: U$1.6 26.46,27.73 25.15,26.42 21.59,26.42 20.57,25.4 17.78,25.4 16.76,24.38 13.63,24.38 R4.2
N$10
  Top 0.254: U$1.23 40.44,36.27 41.15,35.56 41.15,31.24 48.51,23.88 49.87,23.88 R26.2
N$11
  Top 0.254: U$1.41 25.46,41.59 27.69,43.81 U$14.14
N$12
  Top 0.254: U$1.24 33.96,37.01 34.29,37.34 40.13,37.34 41.66,35.81 41.66,31.5 48.77,24.38 51.65,24.38 R27.2
N$13
  Top 0.254: U$1.25 33.46,37.27 34.04,37.85 40.39,37.85 42.16,36.07 42.16,31.75 49.02,24.89 53.43,24.89 R28.2
N$14
  Top 0.254: U$1.5 25.96,27.99 24.89,26.92 21.34,26.92 20.32,25.91 17.53,25.91 16.51,24.89 11.85,24.89 R2.2
N$15
  Top 0.254: R52.2 19.47,35.98 19.81,36.32 21.97,36.32 23.11,35.18 24.26,35.18 24.46,35.38 U$1.43 24.46,44.4 27.69,47.62 U$14.11
N$16  (via drill 0.6)
  Top 0.254: U$1.44 23.96,45.17 v24.38,45.59 | v26.92,45.59 27.69,46.35 U$14.12
  Bottom 0.254: v24.38,45.59 v26.92,45.59
N$17
  Top 0.61: R2.1 9.64,20.98 U$5.P$1
N$18
  Top 0.61: R30.2 U$7.P$3
N$19
  Top 0.305: U$3.32 U$3.31
  Top 0.406: C2.2 56.64,45.59 54.61,47.62 PROG1.5 51.93,48.26 U$3.32
N$20
  Top 0.406: U$28.P$2 65.83,55.83 C6.1 65.18,55.78 IC2.1
N$21
  Top 0.254: U$1.8 27.46,27.21 25.65,25.4 22.1,25.4 21.08,24.38 18.2,24.38 R5.2
N$22
  Top 0.254: U$1.10 28.46,26.68 26.16,24.38 22.61,24.38 21.21,22.99 R7.2
N$23
  Top 0.254: U$1.12 29.46,26.16 26.42,23.11 26.07,23.11 R9.2
N$24
  Top 0.254: U$1.14 30.46,22.93 R11.2
N$25
  Top 0.254: 30.46,34.67 U$1.31 | 29.96,34.67 U$1.32 29.96,41.27 U$14.16 | 29.96,34.67 30.46,34.67 | 29.46,34.67 U$1.33 | 29.46,34.67 29.96,34.67 | C18.1 32.26,31.75 30.46,33.55 30.46,34.67 | 29.46,34.67 28.57,34.67 27.81,33.91 | 27.69,33.78 27.81,33.91 | R52.1 21.59,35.18 22.99,33.78 27.69,33.78 | 27.69,33.78 27.81,33.91
N$26
  Top 0.254: U$1.16 31.46,26.29 R18.2
N$27
  Top 0.254: U$1.18 32.46,26.72 34.8,24.38 37.93,24.38 R21.2
N$28
  Top 0.254: U$1.20 33.46,27.25 35.31,25.4 41.49,25.4 R23.2
N$29
  Top 0.254: U$1.22 34.46,27.77 35.81,26.42 45.05,26.42 R25.2
N$30
  Top 0.406: U$3.16 39.35,52.07 38.97,52.45 38.2,53.21 26.42,53.21 25.27,52.07 U$31.2
N$31
  Top 0.61: 15.49,9.65 15.49,18.1 U$8.P$2 16.78,20.98 R5.1 | R30.1 15.49,9.65 | U$18.4 21.5,6.73 19.56,6.73 18.54,7.75 16.13,7.75 15.49,8.38 15.49,9.65
N$32
  Top 0.406: U$3.2 51.6,51.18 59.82,51.18 62.23,51.18 | 62.23,51.18 PROG1.2 | 62.23,51.18 64.52,53.47 71.88,53.47 84.33,53.47 85.72,52.07 LD1.AR
N$33
  Top 0.406: U$3.1 51.97,50.42 57.66,50.42 58.04,50.42 59.69,48.77 PROG1.3
N$34  (via drill 0.6)
  Top 0.406: U$3.12 45.65,50.29 v46.35,50.29
  Bottom 0.406: v46.35,50.29 55.63,50.29 57.15,48.77 PROG1.4
N$35
  Top 0.254: U$22.42 81.6,44.38 79.63,46.35 U$23.13
N$36
  Top 0.406: U$3.7 49.91,55.15 49.91,55.75 51.44,57.28 53.21,57.28 53.47,57.02 54.74,55.63 SN65.P$4
N$37
  Top 0.406: U$3.6 50.63,54.74 SN65.P$1
N$38  (via drill 0.6)
  Top 0.406: U$2.2 7.11,49.33 7.11,50.16 17.78,60.83 47.37,60.83 49.28,58.93 52.2,58.93 | 52.2,58.93 SN65.P$7 | v101.09,54.61 101.09,55.12 95.38,60.83 57.4,60.83 55.5,58.93 52.2,58.93
  Bottom 0.406: U$19.2 101.4,54.3 v101.09,54.61
N$39
  Top 0.406: 53.47,61.72 17.27,61.72 6.35,50.8 U$2.3 | 53.47,61.72 SN65.P$6 | 53.47,61.72 95.76,61.72 106.68,50.8 U$19.3
N$40
  Top 0.406: R29.2 LD1.C
N$41
  Top 0.406: U$3.3 51.23,51.94 61.85,51.94 64.14,54.23 71.88,54.23 84.33,54.23 87.25,57.15 LD1.AX
N$42
  Top 0.406: U$3.15 39.21,53.34 38.57,53.98 27.81,53.98 26.04,53.98 25.4,53.34 21.46,53.34 20.19,52.07 U$31.4
N$44
  Top 0.406: U$3.14 38.94,54.74 27.81,54.74 26.67,55.88 21.46,55.88 20.19,57.15 U$31.1
N$45
  Top 0.406: U$3.13 39.31,55.5 28.19,55.5 26.54,57.15 U$31.8
N$46  (via drill 0.6)
  Top 0.254: U$1.29 31.46,37.12 v30.86,37.72 | R41.2 C3.2 13.84,32 18.67,36.83 21.72,36.83 v22.23,37.34
  Bottom 0.254: v30.86,37.72 22.48,37.72 v22.23,37.34
N$47
  Top 1.27: U$2.5 11.32,57.8 16.64,63.12 96.27,63.12 101.6,57.78 105.16,57.78 107.31,59.94 107.57,60.2 110.87,60.2 111.63,59.44 111.63,45.21 111.51,45.09 110.22,43.8 U$19.5
N$48
  Top 0.305: C4.1 46.13,59.24 Q1.3
  Top 0.406: U$3.10 44.2,54.01 44.2,54.61 45.09,55.5 47.24,55.5 47.75,56.01 47.75,58.42 47.28,58.89 C4.1
N$49
  Top 0.305: Q1.1 38.07,56.84 C5.1
  Top 0.406: U$3.11 40.23,56.84 Q1.1
N$50
  Top 0.61: R17.2 U$4.P$3
N$51
  Top 0.254: R16.1 2.25,21.12 1.78,21.59 1.78,23.88 2.29,24.38 5.33,24.38 6.86,25.91 7.87,26.92 14.1,26.92 14.22,26.92 17.53,30.23 U$6.P$1
  Top 0.61: R16.1 3.06,20.98 U$4.P$2 1.78,18.1 1.78,8.38 2.16,8 5.21,8 8.13,5.08 U$18.1
N$52
  Top 0.61: R13.1 5.06,20.98 U$4.P$1
N$53
  Top 0.61: 20.07,9.65 20.07,18.1 U$9.P$2 21.35,20.98 R7.1 | R31.1 20.07,9.65 | 20.07,9.65 20.07,8.38 20.7,7.75 23.75,7.75 26.42,5.08 U$18.5
N$54
  Top 0.61: R31.2 U$8.P$3
N$55
  Top 0.61: R6.1 18.78,20.98 U$8.P$1
N$56
  Top 0.61: R20.1 14.21,20.98 U$7.P$1
N$57
  Top 0.61: R8.1 23.35,20.98 U$9.P$1
N$58
  Top 0.61: R10.1 27.94,21.25 27.94,21.59 27.92,21.57 U$10.P$1
N$59
  Top 0.61: R12.1 32.5,20.98 U$11.P$1
N$60
  Top 0.61: R28.1 55.36,20.98 U$17.P$1
N$61
  Top 0.61: R19.1 37.07,20.98 U$12.P$1
N$62
  Top 0.61: R22.1 41.64,20.98 U$13.P$1
N$63
  Top 0.61: R24.1 46.21,20.98 U$15.P$1
N$64
  Top 0.61: R26.1 50.78,20.98 U$16.P$1
N$65
  Top 0.61: 52.07,9.65 52.07,18.1 U$17.P$2 53.36,20.98 R27.1 | 52.07,9.65 R38.1 | 52.07,9.65 52.07,6 U$18.12
N$66  (via drill 0.6)
  Top 0.254: U$1.30 30.96,33.81 31.11,33.66 v31.75,33.66 36.87,33.66 C14.1 | R15.2 v12.83,28.19 12.83,29.59 17.14,33.91 22.1,33.91 22.73,33.27 27.94,33.27 28.32,33.66 28.83,33.66 v29.46,33.66 | v12.83,33.91 R55.2
  Bottom 0.254: v29.46,33.66 v31.75,33.66 | v12.83,28.19 v12.83,33.91
N$67  (via drill 0.6)
  Top 0.254: U$1.28 31.96,38.52 v31.88,38.61 | R40.2 C19.2 v20.95,37.72
  Bottom 0.254: v31.88,38.61 21.84,38.61 v20.95,37.72
N$69
  Top 0.61: 47.5,9.65 R37.1 | 47.5,9.65 47.5,18.1 U$16.P$2 48.78,20.98 R25.1 | 47.5,9.65 47.5,5.24 U$18.11
N$70
  Top 0.61: 42.93,9.65 42.93,18.1 U$15.P$2 44.21,20.98 R23.1 | 42.93,9.65 R36.1 | 42.93,9.65 42.93,6.31 U$18.10
N$71
  Top 0.61: U$16.P$3 R38.2
N$72
  Top 0.61: U$17.P$3 R39.2
N$73
  Top 0.61: U$15.P$3 R37.2
N$74
  Top 0.61: R35.1 38.35,9.65 | 38.35,9.65 38.35,18.1 U$13.P$2 39.64,20.98 R21.1 | 38.35,9.65 38.35,7.38 U$18.9
N$75
  Top 0.61: U$13.P$3 R36.2
N$76
  Top 0.61: 33.78,9.65 33.78,18.1 U$12.P$2 35.07,20.98 R18.1 | R34.1 33.78,9.65 | 33.78,9.65 33.78,8.45 U$18.8
N$77
  Top 0.61: U$12.P$3 R35.2
N$78
  Top 0.61: 29.21,9.65 29.21,18.1 U$11.P$2 30.5,20.98 R11.1 | R33.1 29.21,9.65 | 29.21,9.65 29.21,8.38 30.35,7.24 31.5,7.24 U$18.7
N$79
  Top 0.61: 24.64,9.65 24.64,18.1 U$10.P$2 25.92,20.98 R9.1 | R32.1 24.64,9.65 | 24.64,9.65 24.64,8.51 25.91,7.24 28,7.24 U$18.6
N$80
  Top 0.61: U$10.P$3 R33.2
N$81
  Top 0.61: U$11.P$3 R34.2
N$82
  Top 0.61: U$9.P$3 R32.2
N$83
  Top 0.254: U$1.21 33.96,27.51 35.56,25.91 43.27,25.91 R24.2
N$84
  Top 0.254: U$1.19 32.96,26.98 35.05,24.89 39.71,24.89 R22.2
N$85
  Top 0.254: U$20.2 8.1,35.81 R40.1 R55.1
N$86
  Top 0.254: R15.1 R41.1 5.43,30.1 U$21.2
N$87
  Top 0.254: U$1.7 26.96,27.47 25.4,25.91 21.84,25.91 20.83,24.89 18.03,24.89 17.02,23.88 15.41,23.88 R20.2
N$88
  Top 0.254: U$1.9 27.96,26.94 25.91,24.89 22.35,24.89 21.34,23.88 19.98,23.88 R6.2
N$89
  Top 0.254: R8.2 24.55,23.88 26.42,23.88 28.96,26.42 U$1.11
N$90
  Top 0.254: U$1.13 29.96,25.9 28.07,24 R10.2
N$91
  Top 0.254: U$1.15 30.96,24.5 R12.2
N$92
  Top 0.254: U$22.41 82.1,45.15 79.63,47.62 U$23.14
N$93
  Top 0.254: U$1.17 31.96,26.46 34.54,23.88 36.16,23.88 R19.2
N$94
  Top 0.254: R42.2 80.9,35.05 81.1,35.26 U$22.43 81.1,42.34 79.63,43.81 U$23.11
N$95  (via drill 0.6)
  Top 0.254: U$22.44 80.6,41.57 v80.14,42.04 | v80.14,44.58 79.63,45.09 U$23.12
  Bottom 0.254: v80.14,42.04 v80.14,44.58
N$96
  Top 0.254: 87.1,34.54 U$22.31 | 87.1,34.54 86.49,34.54 86.1,34.54 | 86.1,34.54 U$22.33 86.11,37.34 82.68,40.77 82.68,47.12 79.63,50.16 U$23.16 | U$22.32 86.6,34.54 86.1,34.54 | 87.1,34.54 87.1,33.42 88.77,31.75 C9.1 | 86.1,34.54 85.21,33.66 80.64,33.66 80.39,33.91 76.96,33.91 76.11,34.76 R42.1
N$97  (via drill 0.6)
  Top 0.254: C8.1 92.88,33.66 88.27,33.66 87.6,34.32 U$22.30 87.6,38.33 88.65,39.37 88.9,39.37 98.93,39.37 v101.35,36.96 R44.2 | v101.35,31.24 R43.2
  Bottom 0.254: v101.35,36.96 v101.35,31.24
N$98
  Top 0.254: C10.2 R83.2 101.85,29.34 99.31,31.88 99.31,36.32 97.28,38.35 89.15,38.35 88.6,37.8 U$22.28
N$99
  Top 0.254: U$22.23 97.08,36.27 97.79,35.56 97.79,31.75 97.79,28.7 101.6,24.89 104.65,24.89 105.66,23.88 107.19,23.88 107.57,23.5 R70.2
N$100
  Top 0.254: U$22.24 90.6,37.13 90.68,37.21 90.81,37.34 96.77,37.34 98.3,35.81 98.3,32 98.3,28.96 101.85,25.4 104.9,25.4 105.92,24.38 108.97,24.38 109.86,23.5 R71.2
N$101
  Top 0.254: U$22.25 90.1,37.4 90.55,37.85 97.03,37.85 98.81,36.07 98.81,32.38 98.81,29.21 102.11,25.91 105.28,25.91 106.3,24.89 110.74,24.89 112.14,23.5 R72.2
N$102
  Top 0.254: U$22.29 88.1,38.06 88.9,38.86 97.54,38.86 101.35,35.05 R84.2 C11.2
N$103
  Top 0.61: R47.2 U$24.P$3
N$104
  Top 0.61: U$24.P$1 61.71,21.12 R45.1
N$105
  Top 0.254: 59.71,21.12 58.89,21.12 58.42,21.59 58.42,23.75 61.59,26.92 71.37,26.92 74.17,29.72 74.17,30.53 U$26.P$1
  Top 0.61: R46.1 59.71,21.12 U$24.P$2 58.42,18.1 58.42,8.26 58.42,6.2 U$39.1
N$106
  Top 0.254: U$22.2 81.1,28.78 80.77,28.45 76.71,28.45 75.69,27.43 72.64,27.43 71.63,26.42 62.48,26.42 59.56,23.5 R46.2
N$107
  Top 0.254: U$22.3 81.6,28.52 81.03,27.94 76.96,27.94 75.95,26.92 72.9,26.92 71.88,25.91 64.26,25.91 61.85,23.5 R45.2
N$108
  Top 0.254: U$22.4 82.1,28.25 81.28,27.43 77.22,27.43 76.2,26.42 73.15,26.42 72.14,25.4 66.04,25.4 64.14,23.5 R48.2
N$109
  Top 0.61: 62.99,9.65 R47.1 | 62.99,9.65 62.99,10.16 62.99,18.1 U$25.P$2 64.28,21.12 R48.1 | 62.99,9.65 62.99,5.13 U$39.2
N$110
  Top 0.61: R50.2 U$25.P$3
N$111
  Top 0.61: 67.56,9.65 R50.1 | 67.56,9.65 67.56,10.16 67.56,12.83 67.56,18.1 U$27.P$2 68.85,21.12 R51.1 | 67.56,9.65 67.56,6.1 U$39.3
N$112
  Top 0.254: U$22.6 83.1,27.73 81.79,26.42 77.72,26.42 76.71,25.4 73.66,25.4 72.64,24.38 69.6,24.38 68.71,23.5 R51.2
N$113
  Top 0.254: U$22.5 82.6,27.99 81.53,26.92 77.47,26.92 76.45,25.91 73.41,25.91 72.39,24.89 67.82,24.89 66.42,23.5 R49.2
N$114
  Top 0.61: U$25.P$1 66.28,21.12 R49.1
N$115
  Top 0.61: R73.2 U$27.P$3
N$116
  Top 0.254: U$22.8 84.1,27.21 82.3,25.4 78.23,25.4 77.22,24.38 74.17,24.38 73.28,23.5 R53.2
N$117
  Top 0.254: U$22.10 85.1,26.68 82.8,24.38 78.74,24.38 77.85,23.5 R56.2
N$118
  Top 0.254: U$22.12 86.1,26.16 82.93,22.99 82.72,23.11 R58.2
N$119
  Top 0.254: U$22.14 87.1,22.93 R60.2
N$120
  Top 0.254: U$22.16 88.1,26.29 R62.2
N$121
  Top 0.254: U$22.18 89.1,26.85 91.57,24.38 95.25,24.38 96.14,23.5 R65.2
N$122
  Top 0.254: U$22.20 90.1,27.37 92.08,25.4 98.81,25.4 100.71,23.5 R67.2
N$123
  Top 0.254: U$22.22 91.1,27.9 92.58,26.42 99.31,26.42 101.35,24.38 104.39,24.38 105.28,23.5 R69.2
N$124
  Top 0.61: R53.1 73.42,21.12 U$29.P$2 72.14,18.1 72.14,10.54 72.14,10.16 72.14,9.65 R73.1 69.85,5.27 U$39.4
N$125
  Top 0.61: R56.1 77.99,21.12 U$30.P$2 76.71,18.1 76.71,13.21 76.71,10.16 76.71,9.65 R74.1 74.42,5.96 U$39.5
N$126
  Top 0.61: R74.2 U$29.P$3
N$127
  Top 0.61: U$29.P$1 75.42,21.12 R54.1
N$128
  Top 0.61: U$27.P$1 70.85,21.12 R64.1
N$129
  Top 0.61: U$30.P$1 79.99,21.12 R57.1
N$130
  Top 0.61: U$32.P$1 84.57,21.12 R59.1
N$131
  Top 0.61: U$33.P$1 89.14,21.12 R61.1
N$132
  Top 0.61: U$38.P$1 112,21.12 R72.1
N$133
  Top 0.61: U$34.P$1 93.71,21.12 R63.1
N$134
  Top 0.61: U$35.P$1 98.28,21.12 R66.1
N$135
  Top 0.61: U$36.P$1 102.85,21.12 R68.1
N$136
  Top 0.61: U$37.P$1 107.43,21.12 R70.1
N$137
  Top 0.61: R71.1 110,21.12 U$38.P$2 108.71,18.1 108.71,12.95 108.71,9.65 R81.1 103.51,6.73 102.74,6.73 99.69,6.73 U$39.12
N$138
  Top 0.61: R69.1 105.43,21.12 U$37.P$2 104.14,18.1 104.14,13.08 104.14,9.65 R80.1 100.08,7.87 99.57,7.87 97.34,7.87 U$39.11
N$139
  Top 0.61: R67.1 100.85,21.12 U$36.P$2 99.57,18.1 99.57,13.08 99.57,9.65 R79.1 94.87,7.24 93.2,7.24 U$39.10
N$140
  Top 0.61: U$37.P$3 R81.2
N$141
  Top 0.61: U$38.P$3 R82.2
N$142
  Top 0.61: U$36.P$3 R80.2
N$143
  Top 0.61: R65.1 96.28,21.12 U$35.P$2 95,18.1 95,13.97 95,9.65 R78.1 92.11,9.65 U$39.9
N$144
  Top 0.61: U$35.P$3 R79.2
N$145
  Top 0.61: R62.1 91.71,21.12 U$34.P$2 90.42,18.1 90.42,12.19 90.42,10.16 90.42,9.65 R77.1 88.14,9.18 U$39.8
N$146
  Top 0.61: U$34.P$3 R78.2
N$147
  Top 0.61: R60.1 87.14,21.12 U$33.P$2 85.85,18.1 85.85,10.16 85.85,9.65 R76.1 83.57,8.1 U$39.7
N$148
  Top 0.61: R58.1 82.57,21.12 U$32.P$2 81.28,18.1 81.28,16.89 81.28,10.16 81.28,9.65 R75.1 78.99,7.03 U$39.6
N$149
  Top 0.61: U$32.P$3 R76.2
N$150
  Top 0.61: U$33.P$3 R77.2
N$151
  Top 0.61: U$30.P$3 R75.2
N$152
  Top 0.254: U$22.7 83.6,27.47 82.04,25.91 77.98,25.91 76.96,24.89 73.91,24.89 72.9,23.88 71.37,23.88 70.99,23.5 R64.2
N$153
  Top 0.254: U$22.9 84.6,26.94 82.55,24.89 78.49,24.89 77.47,23.88 75.95,23.88 75.56,23.5 R54.2
N$154
  Top 0.254: U$22.11 85.6,26.42 83.06,23.88 80.52,23.88 80.14,23.5 R57.2
N$155
  Top 0.254: U$22.13 86.6,24.71 R59.2
N$156
  Top 0.254: U$22.15 87.6,24.5 R61.2
N$157
  Top 0.254: U$22.17 88.6,26.59 91.31,23.88 93.47,23.88 93.85,23.5 R63.2
N$158
  Top 0.254: U$22.19 89.6,27.11 91.82,24.89 97.03,24.89 98.42,23.5 R66.2
N$159
  Top 0.254: U$22.21 90.6,27.64 92.33,25.91 99.06,25.91 101.09,23.88 102.62,23.88 103,23.5 R68.2
N$160
  Top 0.254: U$40.1 108.11,29.34 R83.1 R43.1
N$161
  Top 0.254: R84.1 R44.1 106.49,38.83 U$41.1
V+
  Top 0.254: C13.1 21.17,30.77 U$6.P$2 23.96,30.61 U$1.1
V+1
  Top 0.254: U$22.1 80.6,30.61 U$26.P$2 77.65,32.89 C7.1
VIA
  Top 0.406: U$3.23 43.98,43.56 42.93,43.56 42.16,44.32 40.13,44.32 39.62,43.81 U$14.3
VIA2
  Top 0.406: U$3.29 51.75,44.2 61.85,44.2 64.26,44.2 67.69,47.62 U$23.3
VIB
  Top 0.406: U$3.22 43.61,44.32 43.31,44.32 42.55,45.09 U$14.4
VIB2
  Top 0.406: U$3.28 51.38,43.43 64.64,43.43 67.56,46.35 U$23.4
VIC
  Top 0.406: U$14.5 41.11,46.35 U$3.18
VIC2
  Top 0.406: U$3.27 51.01,42.67 65.02,42.67 67.44,45.09 U$23.5
VOD
  Top 0.406: U$14.6 41.25,47.62 U$3.17
VOD2
  Top 0.406: U$3.26 50.64,41.91 65.41,41.91 67.31,43.81 U$23.6

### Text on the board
tPlace: STATUS | MODULE ID | GND | GND | ZEVA BMS24 v1.1 (OS Edition) | 24-cell Lithium Battery | Management Module | + | -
